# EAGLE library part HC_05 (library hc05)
HC-05 Bluetooth Module
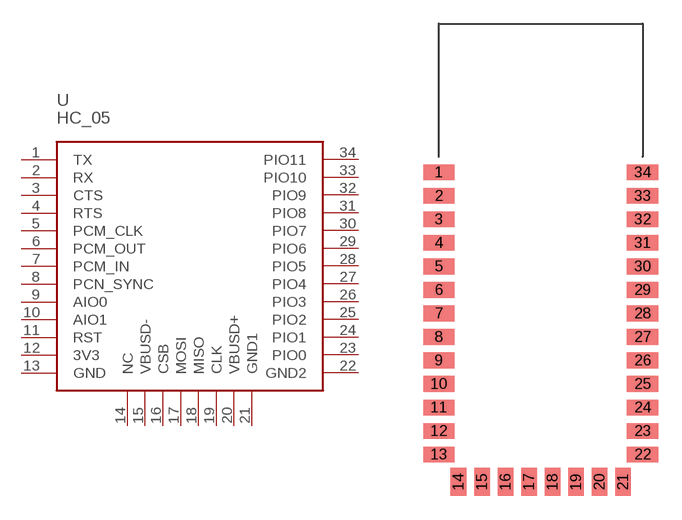
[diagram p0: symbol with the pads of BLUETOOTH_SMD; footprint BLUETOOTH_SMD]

Designator prefix U

## HC_05  [BLUETOOTH_SMD]
1  TX
2  RX
3  CTS
4  RTS
5  PCM_CLK
6  PCM_OUT
7  PCM_IN
8  PCN_SYNC
9  AIO0
10  AIO1
11  RST
12  3V3
13  GND
14  NC
15  VBUSD-
16  CSB
17  MOSI
18  MISO
19  CLK
20  VBUSD+
21  GND1
22  GND2
23  PIO0
24  PIO1
25  PIO2
26  PIO3
27  PIO4
28  PIO5
29  PIO6
30  PIO7
31  PIO8
32  PIO9
33  PIO10
34  PIO11

## Footprint BLUETOOTH_SMD (pad centres in mm)
HC-05
smd 2 x 1: 1 -6.35,3.81; 2 -6.35,2.31; 3 -6.35,0.81; 4 -6.35,-0.69; 5 -6.35,-2.19; 6 -6.35,-3.69; 7 -6.35,-5.19; 8 -6.35,-6.69; 9 -6.35,-8.19; 10 -6.35,-9.69; 11 -6.35,-11.19; 12 -6.35,-12.69; 13 -6.35,-14.19; 22 6.65,-14.19; 23 6.65,-12.69; 24 6.65,-11.19; 25 6.65,-9.69; 26 6.65,-8.19; 27 6.65,-6.69; 28 6.65,-5.19; 29 6.65,-3.69; 30 6.65,-2.19; 31 6.65,-0.69; 32 6.65,0.81; 33 6.65,2.31; 34 6.65,3.81
smd 1 x 1.8: 14 -5.1,-15.94; 15 -3.6,-15.94; 16 -2.1,-15.94; 17 -0.6,-15.94; 18 0.9,-15.94; 19 2.4,-15.94; 20 3.9,-15.94; 21 5.4,-15.94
